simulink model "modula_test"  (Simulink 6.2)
settings: Solver=ode45  StartTime=0.0  StopTime=3  MaxStep=0.001  MinStep=0.0001  RelTol=1e-3

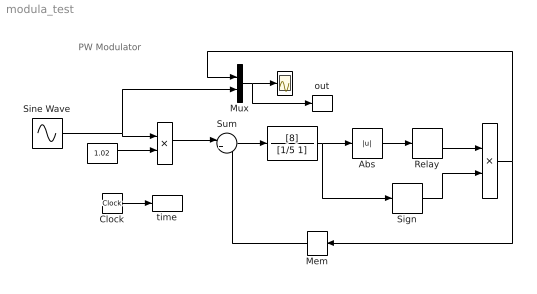
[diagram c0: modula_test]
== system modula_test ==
  note: PW Modulator
  " " : Product
  "  " : TransferFcn  Numerator=[8]  Denominator=[1/5 1]
  "   " : Constant  Value=1.02
  "    " : Product
  "     " : Scope
  Abs : Abs
  Clock : Clock
  Mem : Memory  Orientation=left
  Mux : Mux  Inputs=2
  Relay : Relay  OnSwitchValue=0.5  OffSwitchValue=0.5
  Sign : Signum
  Sine Wave : Sin  Amplitude=0.5  Bias=0.5  Frequency=2  Phase=-1.2  SampleTime=0
  Sum : Sum  Inputs=|+-
  out : ToWorkspace  VariableName=out  SampleTime=-1  SaveFormat=Array
  time : ToWorkspace  VariableName=time  SampleTime=-1  SaveFormat=Array
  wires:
  " "/1 -> Sum/1
  "   "/1 -> " "/2
  Sum/1 -> "  "/1
  "  "/1 -> Abs/1, Sign/1
  Abs/1 -> Relay/1
  Relay/1 -> "    "/1
  Sign/1 -> "    "/2
  Mem/1 -> Sum/2
  "    "/1 -> Mem/1, Mux/1
  Sine Wave/1 -> " "/1, Mux/2
  Mux/1 -> "     "/1, out/1
  Clock/1 -> time/1
